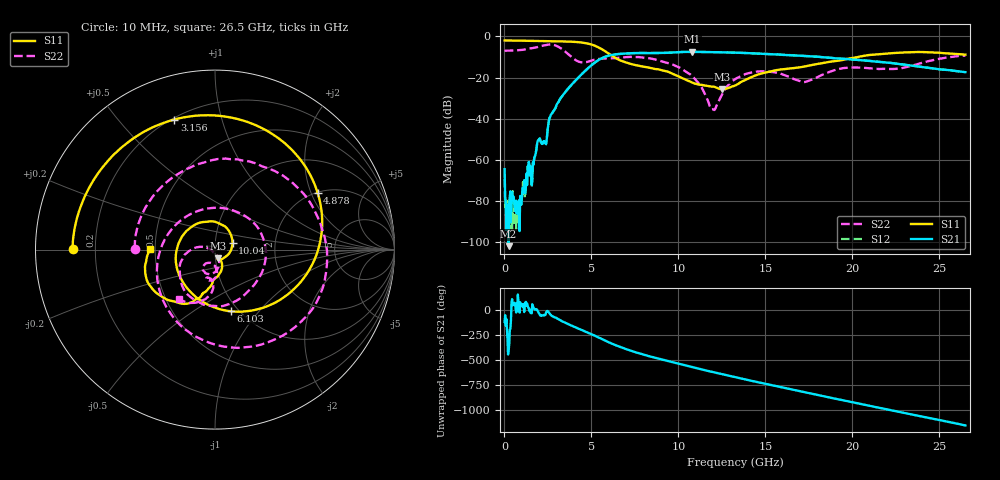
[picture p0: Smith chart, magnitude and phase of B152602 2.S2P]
!  2-Port S-parameters saved by WinCal
! VAR MeasName=S-Parameters (CALIBRATED_DATA) read from VNA (N5242A)
! VAR MeasDate=2016-1-5 16:25:36
! VAR NAME=B152602 2
! VAR FILENAME=B152602 2.S2P
! VAR DATE=2016-1-5 16:25:36
! VAR PHYS_PORTS=1,2
# Hz S DB R 50
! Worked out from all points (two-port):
!   801 points, 10 MHz to 26.5 GHz, reference 50 ohm
!   highest |S21| = -7.52 dB at 10.8 GHz (marker M1); lowest = -101.8 dB at 241.8 MHz (marker M2)
!   |S21| within 3 dB of the highest: 5.625 GHz to 18.84 GHz (13.22 GHz wide, 108 % of centre)
!   lowest |S11| = -25.7 dB at 12.53 GHz (marker M3), VSWR 1.11, Z = 51.3 - j5.08 ohm
!   |S11| at or under -10 dB: 6.284 GHz to 20.34 GHz (14.05 GHz wide, 106 % of centre)
!   |S22| runs from -35.8 to -3.9 dB; largest |S21 - S12| = 0.003
!   S11 on the Smith chart (normalised r, x): 10 MHz: 0.12, +0.00; 3.156 GHz: 0.21, +0.71; 4.878 GHz: 2.02, +2.23; 6.103 GHz: 0.92, -0.72; 10.04 GHz: 1.21, +0.10; 26.5 GHz: 0.47, +0.00
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1e7  -2.01 179.7  -64.44 -120.9  -69.20 -102.4  -6.97 179.4
2.417875e8  -2.02 175.0  -101.80 -37.3  -82.85 -27.2  -6.95 165.1
8.70925e8  -2.09 162.1  -94.50 -27.7  -82.92 41.6  -6.70 126.0
1.764962e9  -2.20 143.2  -57.96 0.9  -57.92 -1.7  -5.48 62.9
2.52655e9  -2.29 125.1  -42.51 -19.4  -42.52 -19.3  -4.02 -7.7
3.155688e9  -2.39 107.4  -31.03 -98.3  -31.06 -98.4  -5.33 -85.3
3.685488e9  -2.54 89.3  -25.12 -144.8  -25.14 -144.8  -8.81 -152.4
4.447075e9  -3.02 55.1  -18.32 158.5  -18.33 158.5  -12.65 105.2
4.877538e9  -3.70 29.0  -14.92 126.3  -14.93 126.5  -12.14 53.0
6.1027e9  -9.01 -75.9  -9.16 27.1  -9.15 27.1  -10.66 -39.1
7.02985e9  -12.79 -161.7  -8.30 -35.1  -8.28 -35.2  -10.06 -75.6
8.851038e9  -16.04 95.2  -8.08 -128.5  -8.09 -128.6  -11.65 -137.2
1.004309e10  -19.50 21.6  -7.67 179.7  -7.66 179.8  -15.06 -168.7
1.080468e10  -22.46 -25.8  -7.52 146.4  -7.52 146.3  -19.39 173.7
1.196361e10  -24.37 -68.5  -7.69 98.3  -7.68 98.1  -35.37 -138.2
1.252652e10  -25.73 -72.5  -7.75 75.7  -7.73 75.6  -27.86 -71.3
1.3255e10  -23.87 -63.6  -7.91 46.8  -7.91 46.8  -20.79 -77.0
1.497685e10  -17.60 -77.6  -8.57 -19.2  -8.53 -19.3  -16.91 -110.4
1.769208e10  -13.85 -96.4  -9.75 -120.3  -9.71 -120.2  -20.99 -91.3
1.957949e10  -11.19 -107.1  -11.00 171.3  -10.96 171.2  -15.33 -95.3
2.209604e10  -8.28 -133.5  -12.84 80.7  -12.78 80.3  -15.87 -103.4
2.65e10  -8.88 179.5  -17.38 -76.3  -17.41 -76.6  -9.34 -125.7
